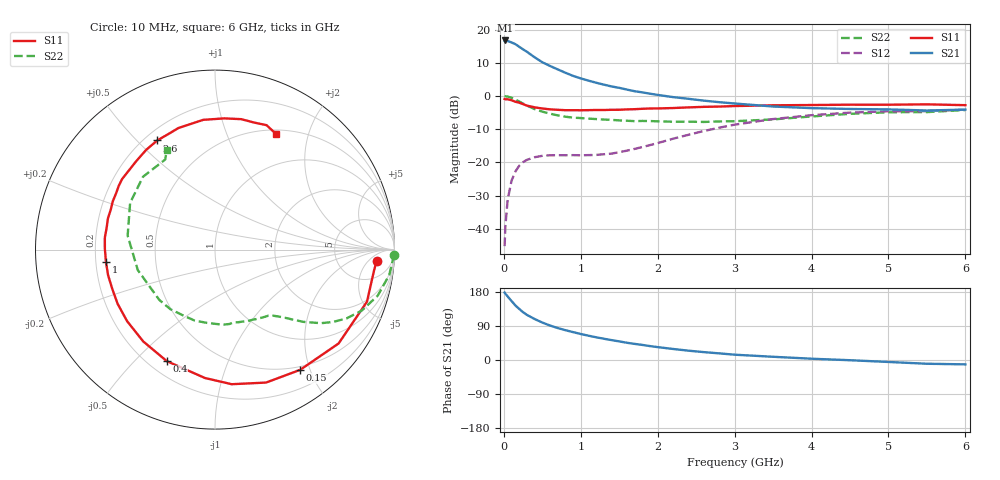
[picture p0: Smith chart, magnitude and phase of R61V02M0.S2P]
! SIEMENS Small Signal Semiconductors
! BFR193
! Si NPN RF Bipolar Junction Transistor in SOT23
! VCE = 1 V  IC = 2 mA
! Common Emitter S-Parameters:  May  1996
# GHz  S  MA  R  50
!  f  S11  S21  S12  S22
! GHz  MAG  ANG  MAG  ANG  MAG  ANG  MAG  ANG
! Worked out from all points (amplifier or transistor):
!   36 points, 10 MHz to 6 GHz, reference 50 ohm
!   highest |S21| = 16.7 dB at 20 MHz (marker M1)
!   |S21| within 3 dB of that: start of sweep to 271.9 MHz
!   unconditionally stable (mu >= 1): 1.14 GHz to 2.209 GHz; 5.366 GHz to end of sweep
!   at 250 MHz: K = 0.24, MSG = 17.0 dB, |S12| = -19.9 dB
!   at 1.4 GHz: K = 1.13, MAG = 7.9 dB, |S12| = -17.3 dB
!   at 6 GHz: K = 1.01, MAG = -0.4 dB, |S12| = -4.1 dB
!   S11 on the Smith chart (normalised r, x): 10 MHz: 14, -9; 150 MHz: 0.45, -1.85; 400 MHz: 0.27, -0.62; 1 GHz: 0.24, -0.05; 2.6 GHz: 0.25, +0.57; 6 GHz: 0.55, +1.51
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0.01  0.9026 -3.9  6.734 177.9  0.0055 87.5  0.9963 -1.6
0.02  0.8932 -7.8  6.869 174.8  0.011 83.9  0.9922 -3.4
0.05  0.8952 -18.9  6.739 167.5  0.0276 80.0  0.9811 -8.3
0.1  0.8648 -37.2  6.412 155.7  0.0531 69.8  0.9422 -15.8
0.15  0.821 -54.7  6.043 143.9  0.0732 61.3  0.8853 -22.6
0.2  0.7935 -69.0  5.516 134.8  0.0892 53.9  0.8272 -27.6
0.25  0.7558 -82.9  5.048 126.1  0.1012 48.1  0.7716 -31.5
0.3  0.7175 -94.5  4.635 119.0  0.1095 43.6  0.7186 -34.8
0.4  0.6769 -113.4  3.836 108.2  0.12 36.8  0.6371 -39.2
0.5  0.6494 -128.0  3.23 98.8  0.126 32.4  0.583 -42.0
0.6  0.6315 -140.9  2.838 91.0  0.1285 29.9  0.5431 -44.3
0.7  0.6208 -151.0  2.521 84.4  0.1287 29.0  0.5117 -46.7
0.8  0.6126 -159.4  2.242 78.7  0.1286 28.9  0.489 -48.8
1  0.6114 -173.6  1.843 68.6  0.1284 30.9  0.4663 -53.4
1.1  0.6136 179.6  1.707 64.1  0.1291 32.9  0.4578 -56.3
1.6  0.6297 154.8  1.251 45.5  0.1508 48.1  0.4251 -72.1
2.2  0.6602 131.5  0.964 29.1  0.228 56.4  0.4108 -96.2
2.6  0.6879 117.9  0.853 20.8  0.2979 54.4  0.4075 -116.1
3.5  0.7259 95.2  0.696 8.5  0.4506 38.9  0.4451 -165.2
4.5  0.7413 78.6  0.639 -0.6  0.5632 19.1  0.54 151.1
5.5  0.7504 67.5  0.606 -9.9  0.5922 1.5  0.5734 118.9
6  0.729 62.2  0.625 -11.5  0.6239 -3.4  0.6163 115.9
